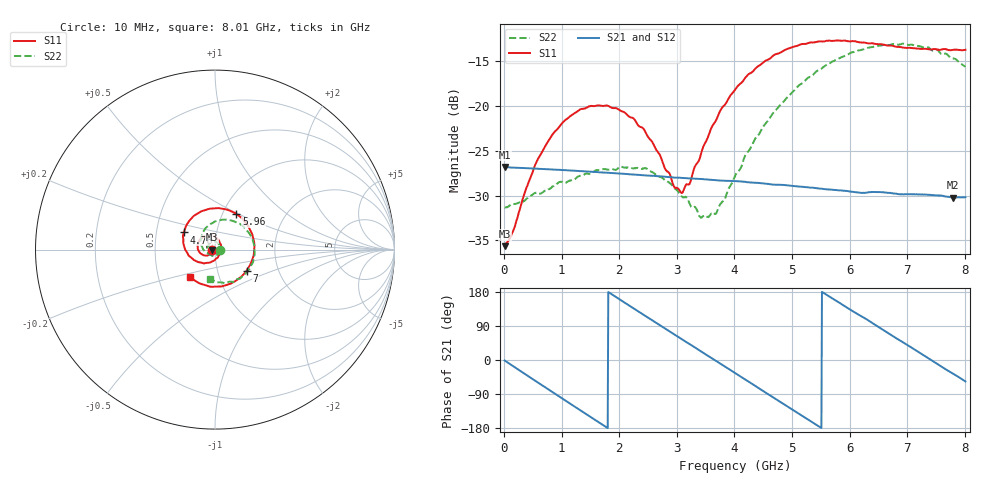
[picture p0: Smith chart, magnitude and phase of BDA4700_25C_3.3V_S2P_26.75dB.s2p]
!Agilent Technologies,E5071B,MY42404982,A.09.10
!Date: Mon Oct 20 18:14:19 2025
!Data & Calibration Information:
!Freq	S11:SOLT2(ON)	S21:SOLT2(ON)	S12:SOLT2(ON)	S22:SOLT2(ON)
# Hz S RI R 50
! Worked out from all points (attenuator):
!   801 points, 10 MHz to 8.01 GHz, reference 50 ohm
!   highest |S21| = -26.81 dB at 10 MHz (marker M1); lowest = -30.2 dB at 7.8 GHz (marker M2)
!   lowest |S11| = -35.7 dB at 10 MHz (marker M3), VSWR 1.03, Z = 48.4 - j0.102 ohm
!   |S11| at or under -10 dB: start of sweep to end of sweep
!   |S22| runs from -32.5 to -13.0 dB; largest |S21 - S12| = 0.0005
!   S11 on the Smith chart (normalised r, x): 10 MHz: 0.97, -0.00; 4.78 GHz: 0.69, +0.14; 5.96 GHz: 1.16, +0.48; 7 GHz: 1.38, -0.34; 8.01 GHz: 0.73, -0.23
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1e7  -0.0165 -0.00106  0.0457 -0.000973  0.0457 -0.000983  0.0271 -0.000811
1.5e8  -0.0174 -0.00945  0.0437 -0.0121  0.0436 -0.012  0.0273 -0.00736
4e8  -0.0259 -0.0244  0.0341 -0.0292  0.0341 -0.0293  0.0215 -0.0217
7e8  -0.0482 -0.0333  0.0147 -0.042  0.0148 -0.0419  0.0062 -0.033
1.03e9  -0.0782 -0.0234  -0.0102 -0.0427  -0.0102 -0.0427  -0.0163 -0.0336
1.35e9  -0.0963 0.00544  -0.0307 -0.0305  -0.0307 -0.0305  -0.0365 -0.0183
2.08e9  -0.0518 0.0768  -0.0372 0.0191  -0.0372 0.0191  -0.0302 0.0338
2.68e9  0.0221 0.0502  -0.00298 0.0404  -0.00305 0.0404  0.0129 0.0383
2.96e9  0.0334 0.0105  0.0154 0.0367  0.0154 0.0367  0.0259 0.0233
3.1e9  0.0309 -0.0111  0.0236 0.0319  0.0234 0.032  0.0287 0.0118
3.23e9  0.0232 -0.0292  0.0296 0.026  0.0297 0.0259  0.0279 0.00287
3.55e9  -0.0168 -0.0662  0.0382 0.00689  0.0382 0.00677  0.0131 -0.02
3.69e9  -0.0417 -0.0733  0.0385 -0.00222  0.0385 -0.00235  0.0015 -0.0253
4.01e9  -0.1052 -0.0641  0.0314 -0.0214  0.0315 -0.0213  -0.031 -0.0259
4.78e9  -0.173 0.0958  -0.0118 -0.0343  -0.0115 -0.0344  -0.078 0.0629
5.35e9  -0.0684 0.2161  -0.0337 -0.00964  -0.0336 -0.00981  -0.0157 0.1469
5.96e9  0.1187 0.1977  -0.0248 0.0226  -0.0249 0.0224  0.1218 0.1508
6.68e9  0.2173 -0.0133  0.0114 0.0307  0.0115 0.0307  0.2195 -6.31e-06
7e9  0.1764 -0.1165  0.0247 0.0207  0.0248 0.0204  0.2033 -0.0851
7.44e9  0.0494 -0.2016  0.0318 -0.00139  0.0318 -0.00136  0.1158 -0.1681
7.8e9  -0.0761 -0.1916  0.0247 -0.0183  0.0247 -0.0184  0.0202 -0.1833
8.01e9  -0.1371 -0.1541  0.0171 -0.0258  0.0171 -0.0257  -0.03 -0.1629
